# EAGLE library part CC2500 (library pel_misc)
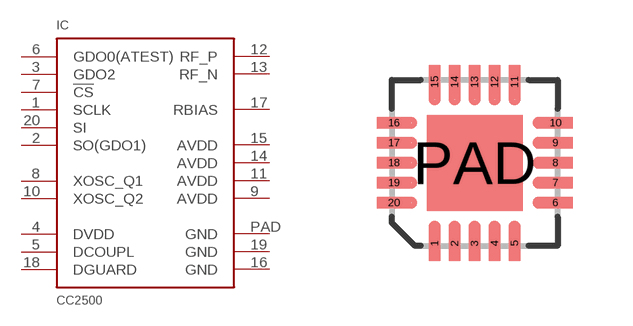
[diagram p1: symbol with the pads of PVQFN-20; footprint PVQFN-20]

Designator prefix IC

## CC2500  [PVQFN-20]
1  SCLK
2  SO(GDO1)
3  GDO2
4  DVDD
5  DCOUPL
6  GDO0(ATEST)
7  !CS
8  XOSC_Q1
9  AVDD
10  XOSC_Q2
11  AVDD
12  RF_P
13  RF_N
14  AVDD
15  AVDD
16  GND
17  RBIAS
18  DGUARD
19  GND
20  SI
PAD  GND

## Footprint PVQFN-20 (pad centres in mm)
smd 0.28 x 0.86: 1 -1,-2.02; 2 -0.5,-2.02; 3 0,-2.02; 4 0.5,-2.02; 5 1,-2.02; 11 1,2.02; 12 0.5,2.02; 13 0,2.02; 14 -0.5,2.02; 15 -1,2.02
smd 0.86 x 0.28: 6 2.02,-1; 7 2.02,-0.5; 8 2.02,0; 9 2.02,0.5; 10 2.02,1; 16 -2.02,1; 17 -2.02,0.5; 18 -2.02,0; 19 -2.02,-0.5; 20 -2.02,-1
smd 2.4 x 2.4: PAD 0,0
